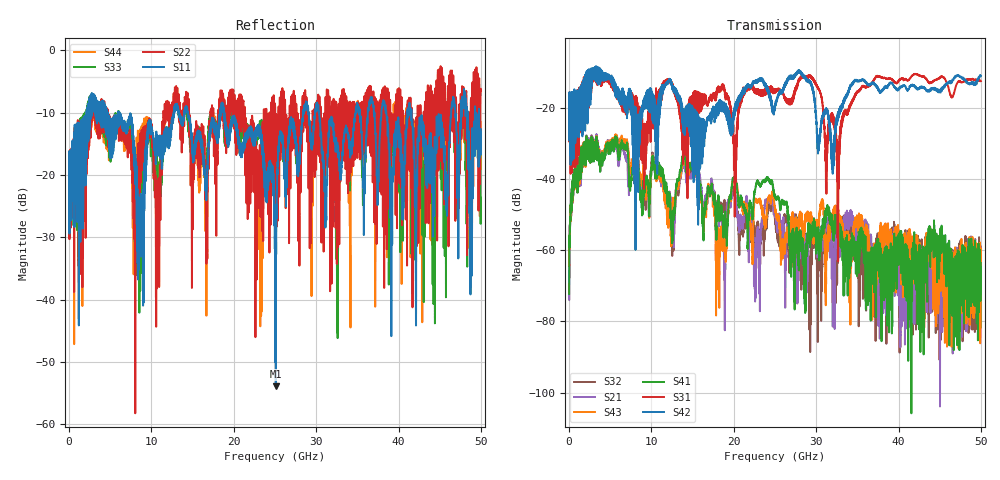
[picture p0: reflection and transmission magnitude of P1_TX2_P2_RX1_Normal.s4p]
!Keysight Technologies,N5225B,MY57041031,A.13.20.10
!Date: Friday, May 31, 2019 11:28:11
!Correction: S11(Full 4 Port(1,2,3,4))
!S12(Full 4 Port(1,2,3,4))
!S13(Full 4 Port(1,2,3,4))
!S14(Full 4 Port(1,2,3,4))
!S21(Full 4 Port(1,2,3,4))
!S22(Full 4 Port(1,2,3,4))
!S23(Full 4 Port(1,2,3,4))
!S24(Full 4 Port(1,2,3,4))
!S31(Full 4 Port(1,2,3,4))
!S32(Full 4 Port(1,2,3,4))
!S33(Full 4 Port(1,2,3,4))
!S34(Full 4 Port(1,2,3,4))
!S41(Full 4 Port(1,2,3,4))
!S42(Full 4 Port(1,2,3,4))
!S43(Full 4 Port(1,2,3,4))
!S44(Full 4 Port(1,2,3,4))
!S4P File: Measurements: <S11,S12,S13,S14>,
!<S21,S22,S23,S24>,
!<S31,S32,S33,S34>,
!<S41,S42,S43,S44>:
# Hz S  dB  R 50.0
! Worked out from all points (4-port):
!   5000 points, 10 MHz to 50 GHz, reference 50 ohm
!   strongest paths, dB at 10 MHz, 12.51 GHz, 25.01 GHz, 37.51 GHz, 50 GHz:
!     S42: -19.3, -14.2, -20.3, -14.7, -11.0
!     S31: -19.4, -13.0, -15.4, -11.1, -12.5
!     S41: -72.3, -55.8, -44.7, -57.9, -71.8
!     S43: -63.4, -49.2, -48.6, -57.7, -64.0
!     S21: -57.4, -47.4, -50.2, -62.5, -66.3
!     S32: -64.4, -55.6, -51.1, -60.3, -66.6
!   lowest |S11| = -53.9 dB at 25.1 GHz (marker M1), VSWR 1.00, Z = 50.1 + j0.193 ohm
!   |S11| at or under -10 dB: 6.091 GHz to 12.71 GHz (6.615 GHz wide, 70.4 % of centre); 18.86 GHz to 28.43 GHz (9.566 GHz wide, 40.5 % of centre); 41.58 GHz to 46.39 GHz (4.81 GHz wide, 10.9 % of centre)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
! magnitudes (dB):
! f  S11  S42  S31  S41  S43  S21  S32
! 10 MHz  -19.8  -19.3  -19.4  -72.3  -63.4  -57.4  -64.4
! 2.01 GHz  -21.7  -21.4  -21.7  -30.4  -30.6  -30.3  -30.5
! 25.1 GHz  -53.9  -18.8  -15.1  -45.3  -50.1  -50.8  -52.8
! 31.66 GHz  -11.9  -25.8  -24.5  -50.0  -56.7  -59.4  -51.5
! 32.64 GHz  -15.8  -21.9  -37.7  -53.5  -48.2  -54.8  -60.2
! 33.37 GHz  -13.7  -17.9  -22.3  -66.5  -54.8  -51.7  -52.9
! 50 GHz  -12.7  -11.0  -12.5  -71.8  -64.0  -66.3  -66.6
